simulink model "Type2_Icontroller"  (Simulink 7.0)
settings: Solver=ode45  StartTime=0.0  StopTime=10.0  RelTol=1e-3
undefined symbols (not defined in the file or in its folder): plecs

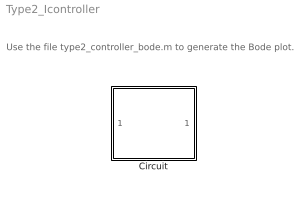
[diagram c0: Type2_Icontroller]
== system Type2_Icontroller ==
  note: Use the file type2_controller_bode.m to generate the Bode plot.
  Circuit : Subsystem  LoadFcn=plecs('sl', 200);  InitFcn=plecs('sl', 214);  StartFcn=plecs('sl', 208);  StopFcn=plecs('sl', 209);  mask(PlecsCircuit){PLECSData=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}
      mask prompts: PLECSData "PLECS Data (Do not delete or modify!)"
      mask init:
      | % PLACE CUSTOM INITIALIZATIONS ABOVE
      | % DO NOT REMOVE
      | plecs('sl', 215);
      | % DO NOT REMOVE

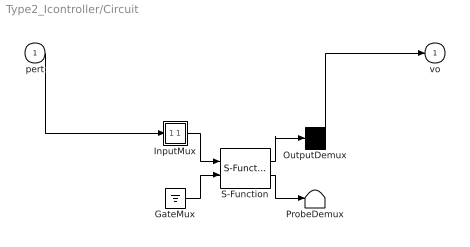
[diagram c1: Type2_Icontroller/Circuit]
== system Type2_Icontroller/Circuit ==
  pert : Inport  PortDimensions=1  OutDataType=sfix(16)  OutScaling=2^0
  " GateMux " : Ground
  " InputMux " : Subsystem
  " OutputDemux " : Demux  Outputs=[ 1 ]
  " ProbeDemux " : Terminator
  " S-Function " : S-Function  FunctionName=plecs
  vo : Outport  PortDimensions=1  OutDataType=sfix(16)  OutScaling=2^0
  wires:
  " S-Function "/1 -> " OutputDemux "/1
  " InputMux "/1(Out) -> " S-Function "/1
  " GateMux "/1 -> " S-Function "/2
  " S-Function "/2 -> " ProbeDemux "/1
  pert/1 -> " InputMux "/1(In1)
  " OutputDemux "/1 -> vo/1

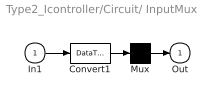
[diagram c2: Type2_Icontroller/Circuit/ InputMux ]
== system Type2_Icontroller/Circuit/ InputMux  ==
  In1 : Inport  OutDataType=sfix(16)  OutScaling=2^0
  Convert1 : DataTypeConversion  OutDataType=sfix(16)  OutScaling=2^0
  Mux : Mux  Inputs=[ 1 ]
  Out : Outport  OutDataType=sfix(16)  OutScaling=2^0
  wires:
  Mux/1 -> Out/1
  In1/1 -> Convert1/1
  Convert1/1 -> Mux/1
